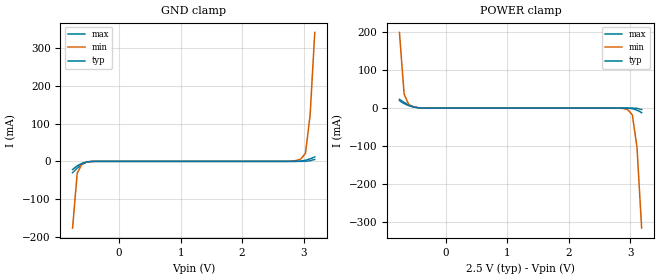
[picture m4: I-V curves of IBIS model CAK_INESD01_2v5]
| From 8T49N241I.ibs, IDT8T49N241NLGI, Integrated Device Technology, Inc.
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| 3.18182e+00   -1.20375e-02   -3.62931e-01   -3.86078e-03
| 3.25758e+00   -2.26391e-02   -5.75917e-01   -1.12361e-02
| 3.33333e+00   -6.36215e-02   -7.89390e-01   -2.21767e-02
| 3.40909e+00   -3.09750e-01   -1.00323e+00   -3.46816e-02
| 3.48485e+00   -5.95739e-01   -1.21733e+00   -4.68684e-02
| 3.56061e+00   -8.82079e-01   -1.43165e+00   -1.11699e-01
| 3.63636e+00   -1.16874e+00   -1.64617e+00   -4.64473e-01
| 3.71212e+00   -1.45569e+00   -1.86086e+00   -8.31334e-01
| 3.78788e+00   -1.74291e+00   -2.07573e+00   -1.19853e+00
| 3.86364e+00   -2.03038e+00   -2.29077e+00   -1.56602e+00
| 3.93939e+00   -2.31808e+00   -2.50596e+00   -1.93376e+00
| 4.01515e+00   -2.60599e+00   -2.72131e+00   -2.30173e+00
| 4.09091e+00   -2.89408e+00   -2.93680e+00   -2.66988e+00
| 4.16667e+00   -3.18234e+00   -3.15243e+00   -3.03820e+00
| 4.24242e+00   -3.47074e+00   -3.36819e+00   -3.40665e+00
| 4.31818e+00   -3.75929e+00   -3.58407e+00   -3.77522e+00
| 4.39394e+00   -4.04795e+00   -3.80008e+00   -4.14390e+00
| 4.46970e+00   -4.33672e+00   -4.01620e+00   -4.51267e+00
| 4.54545e+00   -4.62558e+00   -4.23242e+00   -4.88152e+00
| 4.62121e+00   -4.91454e+00   -4.44874e+00   -5.25044e+00
| 4.69697e+00   -5.20356e+00   -4.66515e+00   -5.61943e+00
| 4.77273e+00   -5.49265e+00   -4.88166e+00   -5.98846e+00
| 4.84848e+00   -5.78180e+00   -5.09824e+00   -6.35753e+00
| 4.92424e+00   -6.07101e+00   -5.31491e+00   -6.72663e+00
| 5.00000e+00   -6.36025e+00   -5.53164e+00   -7.09574e+00
[Model] CAK_INESD01_2v5
Model_type   Input
Polarity   Non-Inverting
Vinl = 0.7V
Vinh = 1.7V
|   typ   min   max
C_comp   2pF   1.5pF   2.5pF
|   typ   min   max
[Voltage range]   2.5V   2.375V   2.625V
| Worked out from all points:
|   GND clamp passes 1 mA (typ) near -0.50 V on its own axis
|   POWER clamp passes 1 mA (typ) near -0.46 V on its own axis
[GND_clamp]
|Voltage   I (typ)   I (min)   I (max)
|Note, modeling breaks down at 250mA and above.  This is well beyond the functional   |
|operating range of the device.  Should this scenario occur, catastrophic failure and   |
|possible damage to the device and/or board is of higher concern than the I-V curve   |
|behavior.  The IBIS checker will flag currents in excess of 10A with warnings.  Lines   |
|with currents in excess of 0.35 A have been commented out.  The points still remain|
|available to the user if the user desires to use them.   |
|-2.50000e+00   -6.31272e+00   -5.12654e+00   -7.65728e+00
|-2.42424e+00   -6.02348e+00   -4.90993e+00   -7.28814e+00
|-2.34848e+00   -5.73428e+00   -4.69340e+00   -6.91901e+00
|-2.27273e+00   -5.44513e+00   -4.47695e+00   -6.54991e+00
|-2.19697e+00   -5.15604e+00   -4.26060e+00   -6.18082e+00
|-2.12121e+00   -4.86701e+00   -4.04434e+00   -5.81177e+00
|-2.04545e+00   -4.57807e+00   -3.82819e+00   -5.44276e+00
|-1.96970e+00   -4.28920e+00   -3.61215e+00   -5.07380e+00
|-1.89394e+00   -4.00043e+00   -3.39622e+00   -4.70491e+00
|-1.81818e+00   -3.71177e+00   -3.18041e+00   -4.33609e+00
|-1.74242e+00   -3.42324e+00   -2.96474e+00   -3.96736e+00
|-1.66667e+00   -3.13483e+00   -2.74920e+00   -3.59872e+00
|-1.59091e+00   -2.84658e+00   -2.53381e+00   -3.23020e+00
|-1.51515e+00   -2.55849e+00   -2.31856e+00   -2.86179e+00
|-1.43939e+00   -2.27059e+00   -2.10347e+00   -2.49353e+00
|-1.36364e+00   -1.98290e+00   -1.88855e+00   -2.12544e+00
|-1.28788e+00   -1.69544e+00   -1.67379e+00   -1.75755e+00
|-1.21212e+00   -1.40822e+00   -1.45921e+00   -1.38989e+00
|-1.13636e+00   -1.12128e+00   -1.24483e+00   -1.02250e+00
|-1.06061e+00   -8.34620e-01   -1.03065e+00   -6.55423e-01
|-9.84848e-01   -5.48283e-01   -8.16712e-01   -2.88690e-01
|-9.09091e-01   -2.62296e-01   -6.03100e-01   -6.18054e-02
|-8.33333e-01   -5.02557e-02   -3.89957e-01   -4.19365e-02
-757.6mV  -21.75mA   -176.8mA   -30.27mA
-681.8mV  -11.92mA   -31.42mA   -17.96mA
-606.1mV  -5.225mA   -6.638mA   -8.107mA
-530.3mV  -1.487mA   -1.607mA   -2.246mA
-378.8mV  -25.75uA   -53.93uA   -24.13uA
2.727V    375.4nA    100.9uA    84.96pA
2.879V    106.8uA    2.187mA    552.6nA
2.955V    792.8uA    6.111mA    14.78uA
3.03V     2.866mA    21.14mA    228.9uA
3.106V    6.546mA    121.9mA    1.635mA
3.182V    11.87mA    341.6mA    5.025mA
| 3.25758e+00   1.96321e-02   5.60094e-01   1.03978e-02
| 3.33333e+00   4.87341e-02   7.78554e-01   1.76586e-02
| 3.40909e+00   2.77089e-01   9.97183e-01   2.56603e-02
| 3.48485e+00   5.68769e-01   1.21602e+00   3.28270e-02
| 3.56061e+00   8.60711e-01   1.43506e+00   7.83184e-02
| 3.63636e+00   1.15294e+00   1.65432e+00   4.20952e-01
| 3.71212e+00   1.44546e+00   1.87380e+00   7.94407e-01
| 3.78788e+00   1.73826e+00   2.09348e+00   1.16822e+00
| 3.86364e+00   2.03134e+00   2.31338e+00   1.54240e+00
| 3.93939e+00   2.32470e+00   2.53350e+00   1.91692e+00
| 4.01515e+00   2.61833e+00   2.75382e+00   2.29178e+00
| 4.09091e+00   2.91222e+00   2.97435e+00   2.66697e+00
| 4.16667e+00   3.20638e+00   3.19510e+00   3.04248e+00
| 4.24242e+00   3.50078e+00   3.41605e+00   3.41830e+00
| 4.31818e+00   3.79544e+00   3.63722e+00   3.79442e+00
| 4.39394e+00   4.09035e+00   3.85860e+00   4.17082e+00
| 4.46970e+00   4.38551e+00   4.08019e+00   4.54751e+00
| 4.54545e+00   4.68090e+00   4.30200e+00   4.92447e+00
| 4.62121e+00   4.97653e+00   4.52403e+00   5.30170e+00
| 4.69697e+00   5.27241e+00   4.74629e+00   5.67919e+00
| 4.77273e+00   5.56852e+00   4.96876e+00   6.05694e+00
| 4.84848e+00   5.86487e+00   5.19147e+00   6.43493e+00
| 4.92424e+00   6.16146e+00   5.41442e+00   6.81318e+00
| 5.00000e+00   6.45829e+00   5.63760e+00   7.19167e+00
[Power_clamp]
|Voltage   I (typ)   I (min)   I (max)
|Note, modeling breaks down at 250mA and above.  This is well beyond the functional   |
|operating range of the device.  Should this scenario occur, catastrophic failure and   |
|possible damage to the device and/or board is of higher concern than the I-V curve   |
|behavior.  The IBIS checker will flag currents in excess of 10A with warnings.  Lines   |
|with currents in excess of 0.35 A have been commented out.  The points still remain|
|available to the user if the user desires to use them.   |
|-2.50000e+00   6.45829e+00   5.26948e+00   7.81670e+00
|-2.42424e+00   6.16146e+00   5.04669e+00   7.43781e+00
|-2.34848e+00   5.86487e+00   4.82413e+00   7.05917e+00
|-2.27273e+00   5.56852e+00   4.60180e+00   6.68076e+00
|-2.19697e+00   5.27241e+00   4.37969e+00   6.30261e+00
|-2.12121e+00   4.97653e+00   4.15780e+00   5.92470e+00
|-2.04545e+00   4.68090e+00   3.93613e+00   5.54704e+00
|-1.96970e+00   4.38551e+00   3.71468e+00   5.16964e+00
|-1.89394e+00   4.09035e+00   3.49344e+00   4.79251e+00
|-1.81818e+00   3.79544e+00   3.27241e+00   4.41564e+00
|-1.74242e+00   3.50078e+00   3.05159e+00   4.03905e+00
|-1.66667e+00   3.20638e+00   2.83098e+00   3.66274e+00
|-1.59091e+00   2.91222e+00   2.61058e+00   3.28673e+00
|-1.51515e+00   2.61833e+00   2.39040e+00   2.91102e+00
|-1.43939e+00   2.32470e+00   2.17042e+00   2.53562e+00
|-1.36364e+00   2.03134e+00   1.95066e+00   2.16054e+00
|-1.28788e+00   1.73826e+00   1.73111e+00   1.78580e+00
|-1.21212e+00   1.44546e+00   1.51178e+00   1.41140e+00
|-1.13636e+00   1.15294e+00   1.29266e+00   1.03735e+00
|-1.06061e+00   8.60711e-01   1.07375e+00   6.63656e-01
|-9.84848e-01   5.68769e-01   8.55052e-01   2.90327e-01
|-9.09091e-01   2.77089e-01   6.36541e-01   4.67878e-02
|-8.33333e-01   4.87341e-02   4.18109e-01   3.00573e-02
-757.6mV  19.63mA    199mA      22.98mA
-681.8mV  11.87mA    37mA       14.92mA
-606.1mV  6.546mA    8.97mA     8.294mA
-530.3mV  2.866mA    3.16mA     3.61mA
-303mV    8.428uA    25.32uA    5.206uA
2.803V    -1.864uA   -178.3uA   -2.484nA
2.955V    -244.9uA   -4.054mA   -3.17uA
3.03V     -1.487mA   -17.6mA    -63.94uA
3.106V    -5.225mA   -102.4mA   -675.5uA
3.182V    -11.92mA   -315.5mA   -3.788mA
